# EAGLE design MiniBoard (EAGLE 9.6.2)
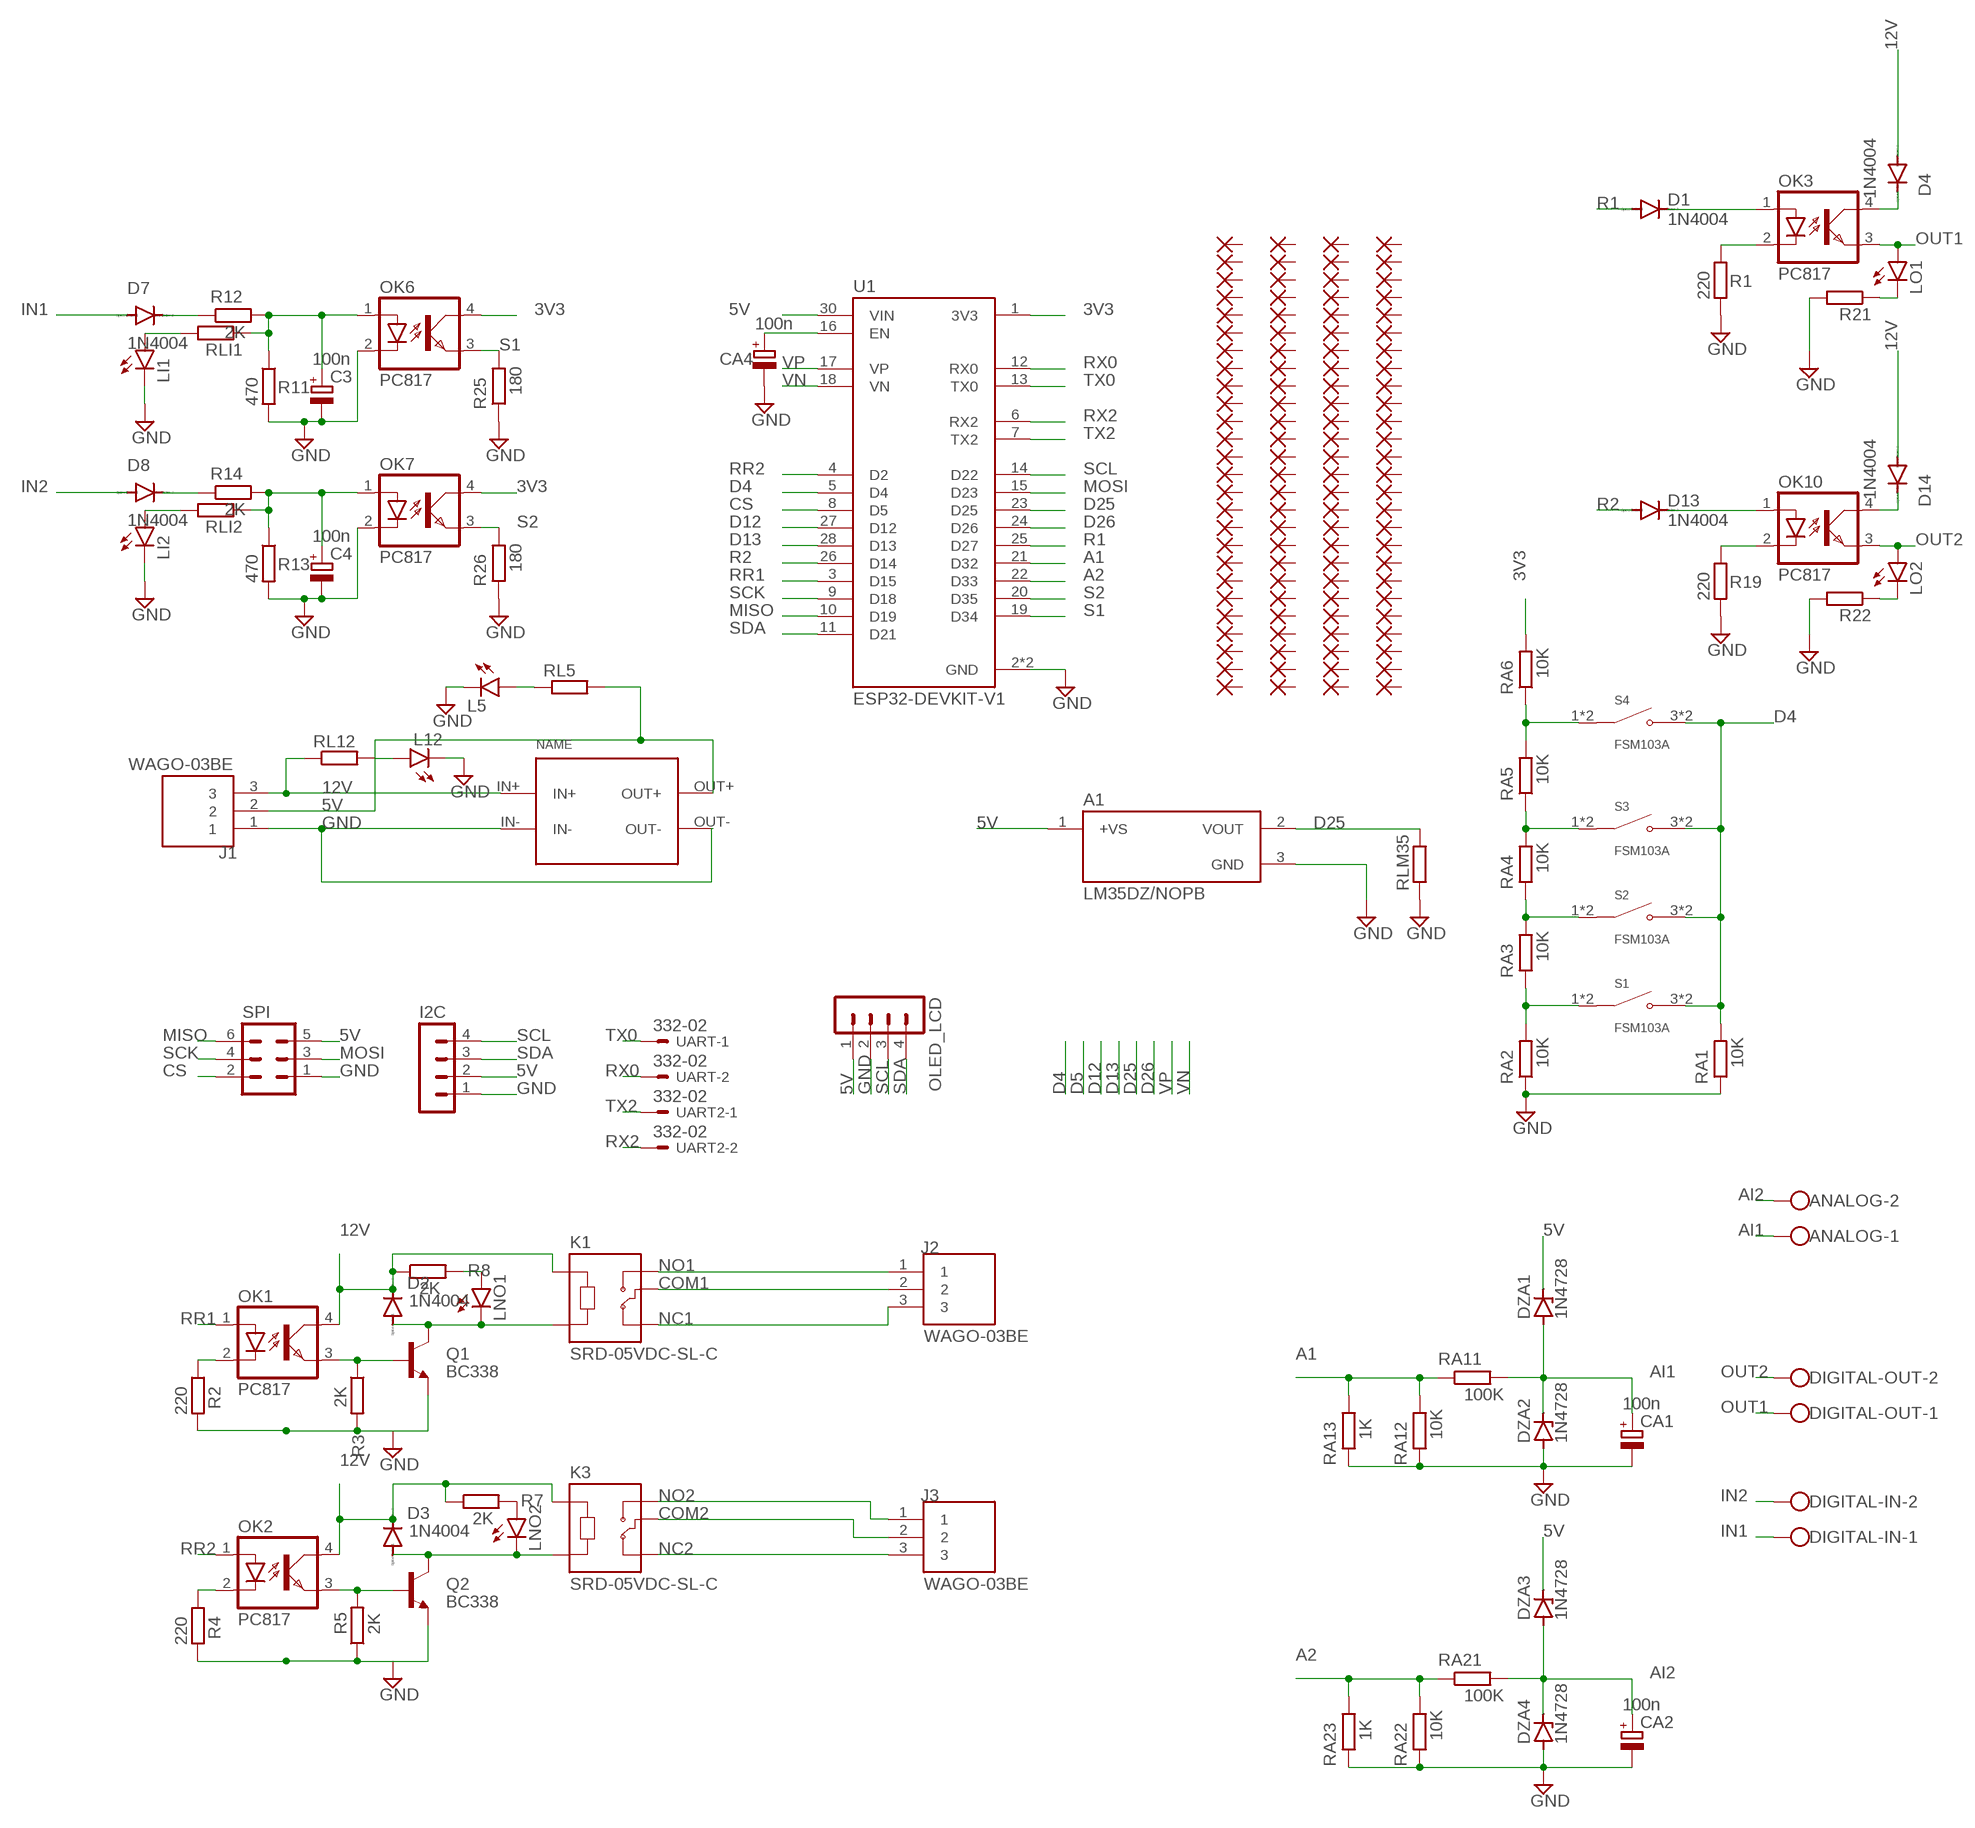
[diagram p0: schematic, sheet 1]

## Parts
A1  LM35DZ/NOPB  [TO92127P521H735-3]
ANALOG  W237-102  [W237-102]
C3  100n  CPOL-EUE5-6  [E5-6]
C4  100n  CPOL-EUE5-6  [E5-6]
CA1  100n  CPOL-EUE5-6  [E5-6]
CA2  100n  CPOL-EUE5-6  [E5-6]
CA4  100n  CPOL-EUE5-6  [E5-6]
D1  1N4004  [DO41-10]
D2  1N4004  [DO41-10]
D3  1N4004  [DO41-10]
D4  1N4004  [DO41-10]
D7  1N4004  [DO41-10]
D8  1N4004  [DO41-10]
D13  1N4004  [DO41-10]
D14  1N4004  [DO41-10]
DIGITAL-IN  W237-102  [W237-102]
DIGITAL-OUT  W237-102  [W237-102]
DZA1  1N4728  [DO41Z10]
DZA2  1N4728  [DO41Z10]
DZA3  1N4728  [DO41Z10]
DZA4  1N4728  [DO41Z10]
I2C  MA04-1  [MA04-1]
J1  WAGO-03BE  [CUI_TB006-508-03BE]
J2  WAGO-03BE  [CUI_TB006-508-03BE]
J3  WAGO-03BE  [CUI_TB006-508-03BE]
K1  SRD-05VDC-SL-C  [RELAY_SRD-05VDC-SL-C]
K3  SRD-05VDC-SL-C  [RELAY_SRD-05VDC-SL-C]
L5  LED3MM  [LED3MM]
L12  LED3MM  [LED3MM]
LI1  LED3MM  [LED3MM]
LI2  LED3MM  [LED3MM]
LNO1  LED3MM  [LED3MM]
LNO2  LED3MM  [LED3MM]
LO1  LED3MM  [LED3MM]
LO2  LED3MM  [LED3MM]
OK1  PC817  [DIL04]
OK2  PC817  [DIL04]
OK3  PC817  [DIL04]
OK6  PC817  [DIL04]
OK7  PC817  [DIL04]
OK10  PC817  [DIL04]
OLED_LCD  MA04-1  [MA04-1]
PAD1  WIREPAD1,6/0,9  [1,6/0,9]
PAD2  WIREPAD1,6/0,9  [1,6/0,9]
PAD3  WIREPAD1,6/0,9  [1,6/0,9]
PAD4  WIREPAD1,6/0,9  [1,6/0,9]
PAD5  WIREPAD1,6/0,9  [1,6/0,9]
PAD6  WIREPAD1,6/0,9  [1,6/0,9]
PAD7  WIREPAD1,6/0,9  [1,6/0,9]
PAD8  WIREPAD1,6/0,9  [1,6/0,9]
PAD9  WIREPAD1,6/0,9  [1,6/0,9]
PAD10  WIREPAD1,6/0,9  [1,6/0,9]
PAD11  WIREPAD1,6/0,9  [1,6/0,9]
PAD12  WIREPAD1,6/0,9  [1,6/0,9]
PAD13  WIREPAD1,6/0,9  [1,6/0,9]
PAD14  WIREPAD1,6/0,9  [1,6/0,9]
PAD15  WIREPAD1,6/0,9  [1,6/0,9]
PAD16  WIREPAD1,6/0,9  [1,6/0,9]
PAD17  WIREPAD1,6/0,9  [1,6/0,9]
PAD18  WIREPAD1,6/0,9  [1,6/0,9]
PAD19  WIREPAD1,6/0,9  [1,6/0,9]
PAD20  WIREPAD1,6/0,9  [1,6/0,9]
PAD21  WIREPAD1,6/0,9  [1,6/0,9]
PAD22  WIREPAD1,6/0,9  [1,6/0,9]
PAD23  WIREPAD1,6/0,9  [1,6/0,9]
PAD24  WIREPAD1,6/0,9  [1,6/0,9]
PAD25  WIREPAD1,6/0,9  [1,6/0,9]
PAD26  WIREPAD1,6/0,9  [1,6/0,9]
PAD27  WIREPAD1,6/0,9  [1,6/0,9]
PAD28  WIREPAD1,6/0,9  [1,6/0,9]
PAD29  WIREPAD1,6/0,9  [1,6/0,9]
PAD30  WIREPAD1,6/0,9  [1,6/0,9]
PAD31  WIREPAD1,6/0,9  [1,6/0,9]
PAD32  WIREPAD1,6/0,9  [1,6/0,9]
PAD33  WIREPAD1,6/0,9  [1,6/0,9]
PAD34  WIREPAD1,6/0,9  [1,6/0,9]
PAD35  WIREPAD1,6/0,9  [1,6/0,9]
PAD36  WIREPAD1,6/0,9  [1,6/0,9]
PAD37  WIREPAD1,6/0,9  [1,6/0,9]
PAD38  WIREPAD1,6/0,9  [1,6/0,9]
PAD39  WIREPAD1,6/0,9  [1,6/0,9]
PAD40  WIREPAD1,6/0,9  [1,6/0,9]
PAD41  WIREPAD1,6/0,9  [1,6/0,9]
PAD42  WIREPAD1,6/0,9  [1,6/0,9]
PAD43  WIREPAD1,6/0,9  [1,6/0,9]
PAD44  WIREPAD1,6/0,9  [1,6/0,9]
PAD45  WIREPAD1,6/0,9  [1,6/0,9]
PAD46  WIREPAD1,6/0,9  [1,6/0,9]
PAD47  WIREPAD1,6/0,9  [1,6/0,9]
PAD48  WIREPAD1,6/0,9  [1,6/0,9]
PAD49  WIREPAD1,6/0,9  [1,6/0,9]
PAD50  WIREPAD1,6/0,9  [1,6/0,9]
PAD51  WIREPAD1,6/0,9  [1,6/0,9]
PAD52  WIREPAD1,6/0,9  [1,6/0,9]
PAD53  WIREPAD1,6/0,9  [1,6/0,9]
PAD54  WIREPAD1,6/0,9  [1,6/0,9]
PAD55  WIREPAD1,6/0,9  [1,6/0,9]
PAD56  WIREPAD1,6/0,9  [1,6/0,9]
PAD57  WIREPAD1,6/0,9  [1,6/0,9]
PAD58  WIREPAD1,6/0,9  [1,6/0,9]
PAD59  WIREPAD1,6/0,9  [1,6/0,9]
PAD60  WIREPAD1,6/0,9  [1,6/0,9]
PAD61  WIREPAD1,6/0,9  [1,6/0,9]
PAD62  WIREPAD1,6/0,9  [1,6/0,9]
PAD63  WIREPAD1,6/0,9  [1,6/0,9]
PAD64  WIREPAD1,6/0,9  [1,6/0,9]
PAD65  WIREPAD1,6/0,9  [1,6/0,9]
PAD66  WIREPAD1,6/0,9  [1,6/0,9]
PAD67  WIREPAD1,6/0,9  [1,6/0,9]
PAD68  WIREPAD1,6/0,9  [1,6/0,9]
PAD69  WIREPAD1,6/0,9  [1,6/0,9]
PAD70  WIREPAD1,6/0,9  [1,6/0,9]
PAD71  WIREPAD1,6/0,9  [1,6/0,9]
PAD72  WIREPAD1,6/0,9  [1,6/0,9]
PAD73  WIREPAD1,6/0,9  [1,6/0,9]
PAD74  WIREPAD1,6/0,9  [1,6/0,9]
PAD75  WIREPAD1,6/0,9  [1,6/0,9]
PAD76  WIREPAD1,6/0,9  [1,6/0,9]
PAD77  WIREPAD1,6/0,9  [1,6/0,9]
PAD78  WIREPAD1,6/0,9  [1,6/0,9]
PAD79  WIREPAD1,6/0,9  [1,6/0,9]
PAD80  WIREPAD1,6/0,9  [1,6/0,9]
PAD81  WIREPAD1,6/0,9  [1,6/0,9]
PAD82  WIREPAD1,6/0,9  [1,6/0,9]
PAD83  WIREPAD1,6/0,9  [1,6/0,9]
PAD84  WIREPAD1,6/0,9  [1,6/0,9]
PAD85  WIREPAD1,6/0,9  [1,6/0,9]
PAD86  WIREPAD1,6/0,9  [1,6/0,9]
PAD87  WIREPAD1,6/0,9  [1,6/0,9]
PAD88  WIREPAD1,6/0,9  [1,6/0,9]
PAD89  WIREPAD1,6/0,9  [1,6/0,9]
PAD90  WIREPAD1,6/0,9  [1,6/0,9]
PAD91  WIREPAD1,6/0,9  [1,6/0,9]
PAD92  WIREPAD1,6/0,9  [1,6/0,9]
PAD93  WIREPAD1,6/0,9  [1,6/0,9]
PAD94  WIREPAD1,6/0,9  [1,6/0,9]
PAD95  WIREPAD1,6/0,9  [1,6/0,9]
PAD96  WIREPAD1,6/0,9  [1,6/0,9]
PAD97  WIREPAD1,6/0,9  [1,6/0,9]
PAD98  WIREPAD1,6/0,9  [1,6/0,9]
PAD99  WIREPAD1,6/0,9  [1,6/0,9]
PAD100  WIREPAD1,6/0,9  [1,6/0,9]
PAD101  WIREPAD1,6/0,9  [1,6/0,9]
PAD102  WIREPAD1,6/0,9  [1,6/0,9]
PAD103  WIREPAD1,6/0,9  [1,6/0,9]
PAD104  WIREPAD1,6/0,9  [1,6/0,9]
Q1  BC338  [TO92-EBC]
Q2  BC338  [TO92-EBC]
R1  220  R-EU_0309/12  [0309/12]
R2  220  R-EU_0309/12  [0309/12]
R3  2K  R-EU_0309/12  [0309/12]
R4  220  R-EU_0309/12  [0309/12]
R5  2K  R-EU_0309/12  [0309/12]
R7  2K  R-EU_0309/12  [0309/12]
R8  2K  R-EU_0309/12  [0309/12]
R11  470  R-EU_0309/12  [0309/12]
R12  2K  R-EU_0309/12  [0309/12]
R13  470  R-EU_0309/12  [0309/12]
R14  2K  R-EU_0309/12  [0309/12]
R19  220  R-EU_0309/12  [0309/12]
R21  R-EU_0309/12  [0309/12]
R22  R-EU_0309/12  [0309/12]
R25  180  R-EU_0309/12  [0309/12]
R26  180  R-EU_0309/12  [0309/12]
RA1  10K  R-EU_0309/12  [0309/12]
RA2  10K  R-EU_0309/12  [0309/12]
RA3  10K  R-EU_0309/12  [0309/12]
RA4  10K  R-EU_0309/12  [0309/12]
RA5  10K  R-EU_0309/12  [0309/12]
RA6  10K  R-EU_0309/12  [0309/12]
RA11  100K  R-EU_0309/12  [0309/12]
RA12  10K  R-EU_0309/12  [0309/12]
RA13  1K  R-EU_0309/12  [0309/12]
RA21  100K  R-EU_0309/12  [0309/12]
RA22  10K  R-EU_0309/12  [0309/12]
RA23  1K  R-EU_0309/12  [0309/12]
RL5  R-EU_0309/12  [0309/12]
RL12  R-EU_0309/12  [0309/12]
RLI1  R-EU_0309/12  [0309/12]
RLI2  R-EU_0309/12  [0309/12]
RLM35  R-EU_0309/12  [0309/12]
S1  FSM103A  [SW_1571627-1]
S2  FSM103A  [SW_1571627-1]
S3  FSM103A  [SW_1571627-1]
S4  FSM103A  [SW_1571627-1]
SPI  MA03-2  [MA03-2]
U1  ESP32-DEVKIT-V1  [MODULE_ESP32_DEVKIT_V1]
U$1  CP8-ADJ  [CP8-ADJ]
UART  332-02  [332-02]
UART2  332-02  [332-02]

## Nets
3V3: OK6.4(COL) OK7.4(COL) RA6.2 U1.1(3V3)
5V: A1.1(+VS) DZA1.C DZA3.C I2C.2 J1.2 OLED_LCD.1 RL5.2 SPI.5 U1.30(VIN) U$1.OUT+
12V: D2.C D3.C D4.A D14.A J1.3 K1.A1 K3.A1 OK1.4(COL) OK2.4(COL) R7.1 R8.1 RL12.1 U$1.IN+
A1: RA11.1 RA12.2 RA13.2 U1.21(D32)
A2: RA21.1 RA22.2 RA23.2 U1.22(D33)
AI1: ANALOG.1 CA1.+ DZA1.A DZA2.C RA11.2
AI2: ANALOG.2 CA2.+ DZA3.A DZA4.C RA21.2
COM1: J2.2 K1.COM
COM2: J3.2 K3.COM
CS: SPI.2 U1.8(D5)
D4: RA1.2 S1.3(NO) S1.4(NO) S2.3(NO) S2.4(NO) S3.3(NO) S3.4(NO) S4.3(NO) S4.4(NO) U1.5(D4)
D12: U1.27(D12)
D13: U1.28(D13)
D25: A1.2(VOUT) RLM35.2 U1.23(D25)
D26: U1.24(D26)
GND: A1.3(GND) C3.- C4.- CA1.- CA2.- CA4.- DZA2.A DZA4.A I2C.1 J1.1 L5.K(C) L12.K(C) LI1.K(C) LI2.K(C) OK6.2(C) OK7.2(C) OLED_LCD.2 Q1.E Q2.E R1.2 R2.2 R3.2 R4.2 R5.1 R11.2 R13.2 R19.2 R21.2 R22.2 R25.1 R26.1 RA1.1 RA2.1 RA12.1 RA13.1 RA22.1 RA23.1 RLM35.1 SPI.1 U1.2(GND) U1.29(GND) U$1.IN- U$1.OUT-
IN1: D7.A DIGITAL-IN.1
IN2: D8.A DIGITAL-IN.2
MISO: SPI.6 U1.10(D19)
MOSI: SPI.3 U1.15(D23)
N$1: OK2.2(C) R4.1
N$2: OK1.2(C) R2.1
N$3: OK1.3(EMIT) Q1.B R3.1
N$4: D3.A K3.A2 LNO2.K(C) Q2.C
N$5: RA4.2 RA5.1 S3.1(COM) S3.2(COM)
N$6: OK2.3(EMIT) Q2.B R5.2
N$7: LNO2.A R7.2
N$8: RA3.2 RA4.1 S2.1(COM) S2.2(COM)
N$9: RA2.2 RA3.1 S1.1(COM) S1.2(COM)
N$10: LNO1.A R8.2
N$11: D2.A K1.A2 LNO1.K(C) Q1.C
N$14: L12.A RL12.2
N$15: D1.C OK3.1(A)
N$16: OK3.2(C) R1.1
N$18: D4.C OK3.4(COL)
N$19: C3.+ OK6.1(A) R11.1 R12.2 RLI1.1
N$20: D7.C R12.1
N$21: C4.+ OK7.1(A) R13.1 R14.2 RLI2.1
N$22: D8.C R14.1
N$23: L5.A RL5.1
N$24: LI2.A RLI2.2
N$25: CA4.+ U1.16(EN)
N$26: D13.C OK10.1(A)
N$27: OK10.2(C) R19.1
N$29: LI1.A RLI1.2
N$30: LO1.K(C) R21.1
N$31: LO2.K(C) R22.1
N$32: RA5.2 RA6.1 S4.1(COM) S4.2(COM)
N$52: D14.C OK10.4(COL)
NC1: J2.3 K1.NC
NC2: J3.3 K3.NC
NO1: J2.1 K1.NO
NO2: J3.1 K3.NO
OUT1: DIGITAL-OUT.1 LO1.A OK3.3(EMIT)
OUT2: DIGITAL-OUT.2 LO2.A OK10.3(EMIT)
R1: D1.A U1.25(D27)
R2: D13.A U1.26(D14)
RR1: OK1.1(A) U1.3(D15)
RR2: OK2.1(A) U1.4(D2)
RX0: U1.12(RX0) UART.2
RX2: U1.6(RX2) UART2.2
S1: OK6.3(EMIT) R25.2 U1.19(D34)
S2: OK7.3(EMIT) R26.2 U1.20(D35)
SCK: SPI.4 U1.9(D18)
SCL: I2C.4 OLED_LCD.3 U1.14(D22)
SDA: I2C.3 OLED_LCD.4 U1.11(D21)
TX0: U1.13(TX0) UART.1
TX2: U1.7(TX2) UART2.1
VN: U1.18(VN)
VP: U1.17(VP)
Unconnected: PAD1.1(P) PAD2.1(P) PAD3.1(P) PAD4.1(P) PAD5.1(P) PAD6.1(P) PAD7.1(P) PAD8.1(P) PAD9.1(P) PAD10.1(P) PAD11.1(P) PAD12.1(P) PAD13.1(P) PAD14.1(P) PAD15.1(P) PAD16.1(P) PAD17.1(P) PAD18.1(P) PAD19.1(P) PAD20.1(P) PAD21.1(P) PAD22.1(P) PAD23.1(P) PAD24.1(P) PAD25.1(P) PAD26.1(P) PAD27.1(P) PAD28.1(P) PAD29.1(P) PAD30.1(P) PAD31.1(P) PAD32.1(P) PAD33.1(P) PAD34.1(P) PAD35.1(P) PAD36.1(P) PAD37.1(P) PAD38.1(P) PAD39.1(P) PAD40.1(P) PAD41.1(P) PAD42.1(P) PAD43.1(P) PAD44.1(P) PAD45.1(P) PAD46.1(P) PAD47.1(P) PAD48.1(P) PAD49.1(P) PAD50.1(P) PAD51.1(P) PAD52.1(P) PAD53.1(P) PAD54.1(P) PAD55.1(P) PAD56.1(P) PAD57.1(P) PAD58.1(P) PAD59.1(P) PAD60.1(P) PAD61.1(P) PAD62.1(P) PAD63.1(P) PAD64.1(P) PAD65.1(P) PAD66.1(P) PAD67.1(P) PAD68.1(P) PAD69.1(P) PAD70.1(P) PAD71.1(P) PAD72.1(P) PAD73.1(P) PAD74.1(P) PAD75.1(P) PAD76.1(P) PAD77.1(P) PAD78.1(P) PAD79.1(P) PAD80.1(P) PAD81.1(P) PAD82.1(P) PAD83.1(P) PAD84.1(P) PAD85.1(P) PAD86.1(P) PAD87.1(P) PAD88.1(P) PAD89.1(P) PAD90.1(P) PAD91.1(P) PAD92.1(P) PAD93.1(P) PAD94.1(P) PAD95.1(P) PAD96.1(P) PAD97.1(P) PAD98.1(P) PAD99.1(P) PAD100.1(P) PAD101.1(P) PAD102.1(P) PAD103.1(P) PAD104.1(P)

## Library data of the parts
A1 = LM35DZ_NOPB:LM35DZ/NOPB; CHECK_PRICES: https://www.snapeda.com/parts/LM35DZ/NOPB/Texas+Instruments/view-part/?ref=eda; DESCRIPTION: 1C high voltage analog temperature sensor, 10 mV/C; DIGIKEY_PART_NUMBER: LM35DZ/NOPB-ND; MF: Texas; MP: LM35DZ/NOPB; PACKAGE: None; SNAPEDA_LINK: https://www.snapeda.com/parts/LM35DZ/NOPB/Texas+Instruments/view-part/?ref=snap
ANALOG DIGITAL-IN DIGITAL-OUT = con-wago-500:W237-102: WAGO SCREW CLAMP; MPN: 237-102; OC_FARNELL: unknown; OC_NEWARK: 70K9898
C3 C4 CA1 CA2 CA4 = rcl-ws:CPOL-EU: POLARIZED CAPACITOR, European symbol; SPICEPREFIX: C
D1-D4 D7 D8 D13 D14 = diode:1N4004: DIODE
DZA1-DZA4 = diode-ws:1N4728: Z DIODE
I2C OLED_LCD = con-lstb:MA04-1: PIN HEADER; OC_FARNELL: unknown; OC_NEWARK: unknown
J1-J3 = TB006-508-03BE:WAGO-03BE: Check availability; AVAILABILITY: In Stock; CHECK_PRICES: https://www.snapeda.com/parts/TB006-508-03BE/Same+Sky/view-part/?ref=eda; DESCRIPTION: 2~24 Poles, Screw Type, Horizontal, 5.08 Pitch, 26~14 (AWG), Terminal Block Connector; MF: Same Sky; MP: TB006-508-03BE; PACKAGE: None; PRICE: None; SNAPEDA_LINK: https://www.snapeda.com/parts/TB006-508-03BE/Same+Sky/view-part/?ref=snap
K1 K3 = SRD-05VDC-SL-C:SRD-05VDC-SL-C: 5V Trigger Relay Module For Arduino And Raspberry Pi 5V Trigger Relay Module For Arduino And Raspberry Pi Check availability; AVAILABILITY: In Stock; CHECK_PRICES: https://www.snapeda.com/parts/SRD-05VDC-SL-C/Songle+Relay/view-part/?ref=eda; DESCRIPTION: 5V Trigger Relay Module For Arduino And Raspberry Pi 5V Trigger Relay Module For Arduino And Raspberry Pi; MF: Songle Relay; MP: SRD-05VDC-SL-C; PACKAGE: NON STANDARD-5 Songle Relay; PRICE: None; SNAPEDA_LINK: https://www.snapeda.com/parts/SRD-05VDC-SL-C/Songle+Relay/view-part/?ref=snap
L5 L12 LI1 LI2 LNO1 LNO2 LO1 LO2 = led_WS:LED: LED
OK1-OK3 OK6 OK7 OK10 = optocoupler:PC817: SHARP OPTO COUPLER; MPN: PC817X4J000F; OC_FARNELL: 9707727; OC_NEWARK: 97K7059
PAD1-PAD104 = wirepad-ws:WIREPAD: Wire PAD connect wire on PCB
Q1 Q2 = transistor-npn:BC338*: NPN Transistor
R1-R5 R7 R8 R11-R14 R19 R21 R22 R25 R26 RA1-RA6 RA11-RA13 RA21-RA23 RL5 RL12 RLI1 RLI2 RLM35 = rcl-ws:R-EU_: RESISTOR, European symbol; SPICEPREFIX: R
S1-S4 = FSM103A:FSM103A: Alcoswitch FSM100-104, Tactile Switches, Round Actuator Style, Operating Function NO, Brass Contact Base Material Check availability; AVAILABILITY: In Stock; CHECK_PRICES: https://www.snapeda.com/parts/FSM103A/TE+Connectivity+ALCOSWITCH+Switches/view-part/?ref=eda; COMMENT: 1571627-1; DESCRIPTION: Alcoswitch, Tactile switch,PCB,SPST,red actuator | TE Connectivity FSM103A; MF: TE Connectivity; MP: FSM103A; PACKAGE: None; PRICE: None; SNAPEDA_LINK: https://www.snapeda.com/parts/FSM103A/TE+Connectivity+ALCOSWITCH+Switches/view-part/?ref=snap
SPI = con-lstb-ws:MA03-2: PIN HEADER; OC_FARNELL: unknown; OC_NEWARK: unknown
U1 = ESP32-DEVKIT-V1:ESP32-DEVKIT-V1: Dual core, Wi-Fi: 2.4 GHz up to 150 Mbits/s,BLE (Bluetooth Low Energy) and legacy Bluetooth, 32 bits, Up to 240 MHz Check availability; AVAILABILITY: Not in stock; CHECK_PRICES: https://www.snapeda.com/parts/ESP32-DEVKIT-V1/Do+it/view-part/?ref=eda; DESCRIPTION: Dual core, Wi-Fi: 2.4 GHz up to 150 Mbits/s,BLE (Bluetooth Low Energy) and legacy Bluetooth, 32 bits, Up to 240 MHz; MF: Do it; MP: ESP32-DEVKIT-V1; PACKAGE: None; PRICE: None; SNAPEDA_LINK: https://www.snapeda.com/parts/ESP32-DEVKIT-V1/Do+it/view-part/?ref=snap
U$1 = userlib:CP8-ADJ: Voltage regulator IN: 7-35V OUT: ADJ
UART UART2 = con-garry-ws:332-02: 2 Pin - 2mm Dual Row

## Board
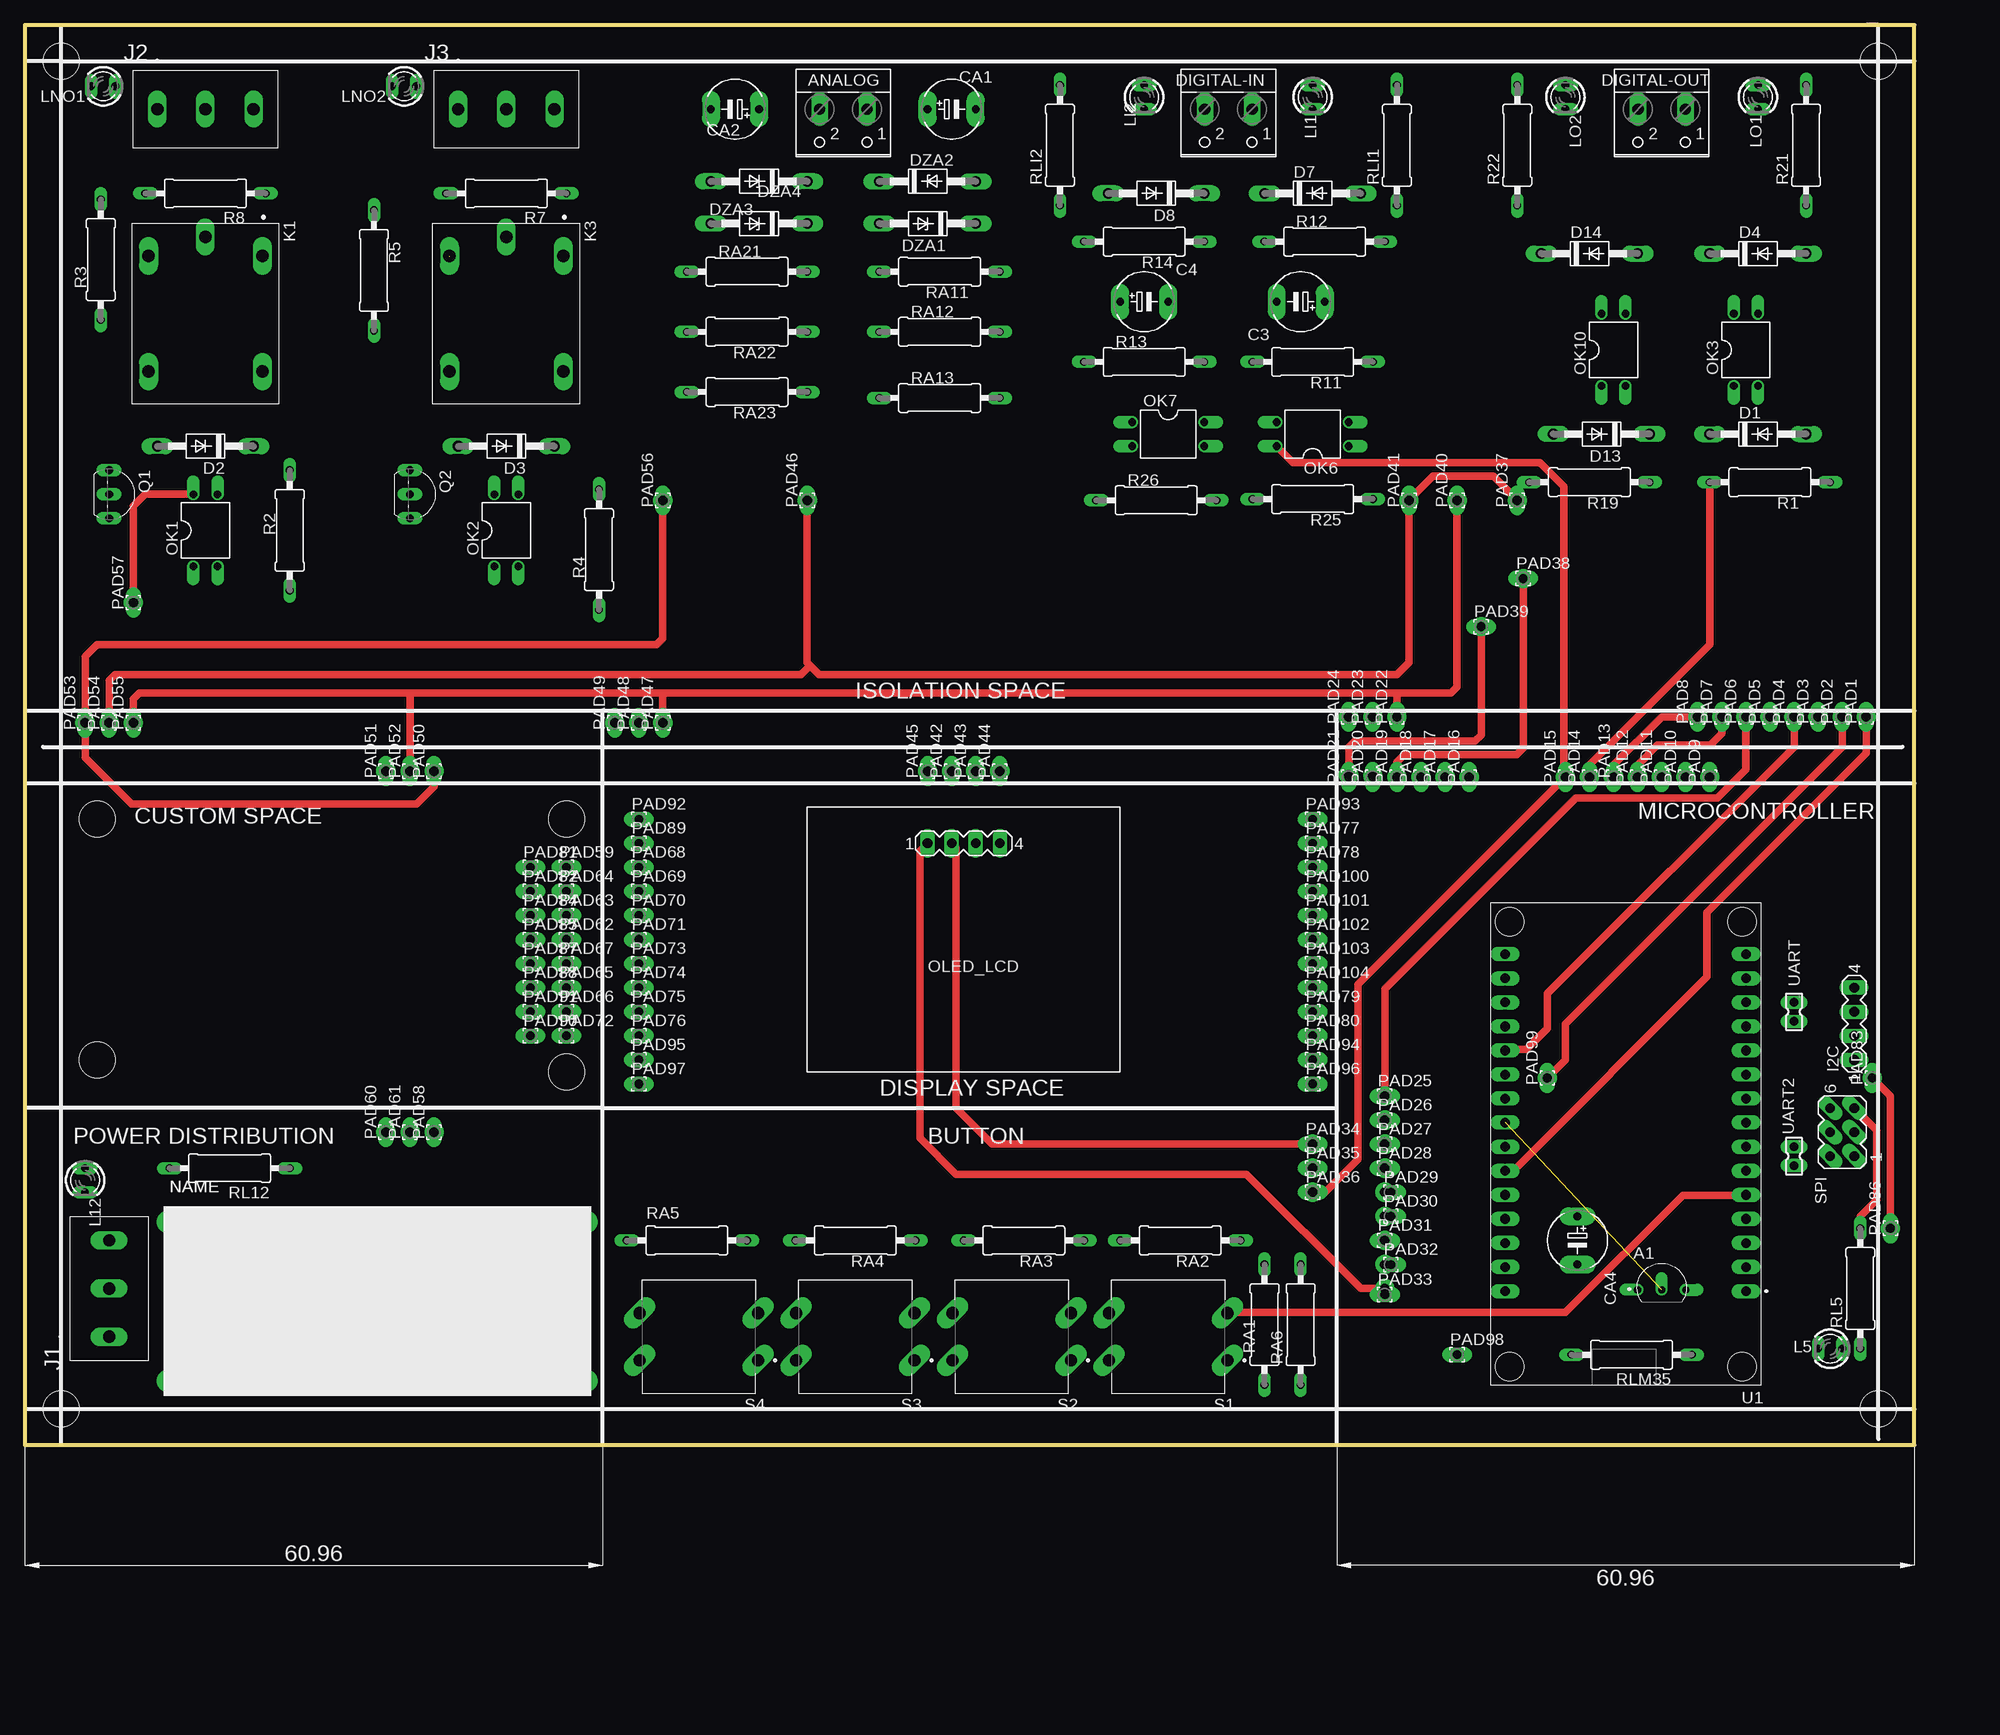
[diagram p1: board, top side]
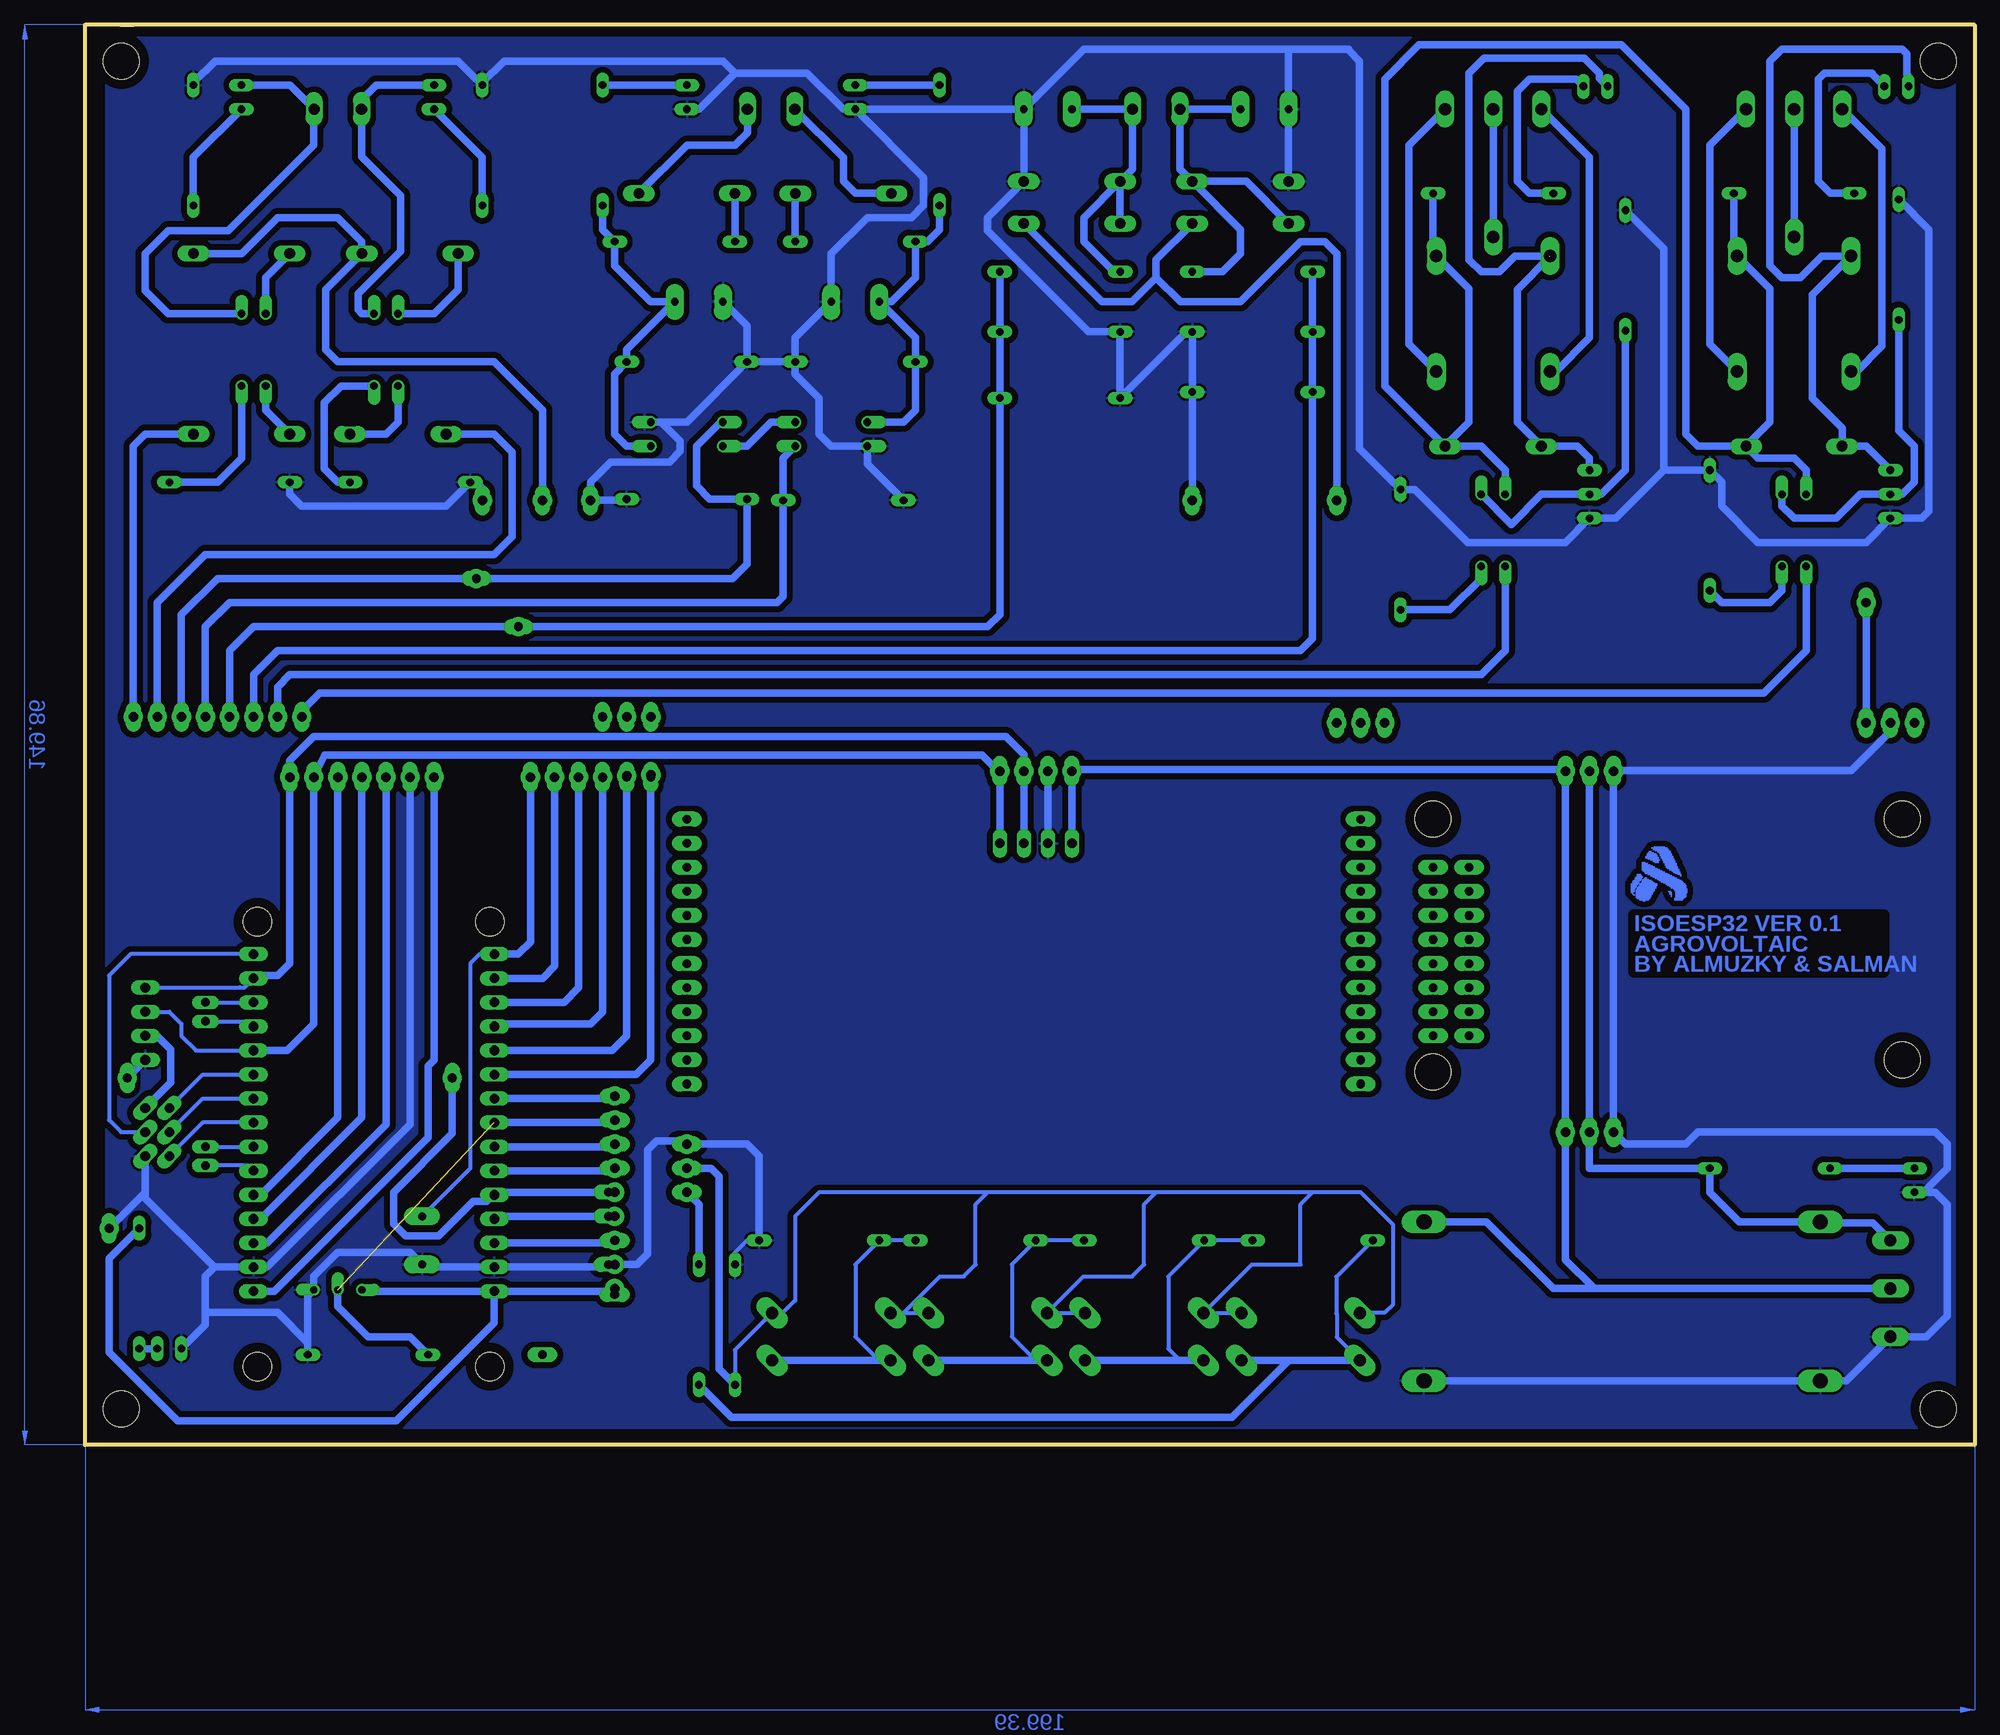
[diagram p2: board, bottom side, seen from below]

Size 199.39 x 149.86 mm. Coordinates in mm from the lower left corner, seen from the top.
Outline: 195.58,149.86 194.31,149.86
Outline: 0,0 199.39,0 199.39,149.86 0,149.86 0,0
Copper layers (1*16): Top 0.035mm / dielectric 1.5mm / Bottom 0.035mm
Design rules "default *": minimum track width 16mil, minimum drill 0.35mm, track to track 24mil, track to pad 24mil, pad to pad 24mil, via to via 6mil, smd to smd 6mil, copper to edge 40mil, drill to drill 6mil, minimum pad ring 10mil, minimum via ring 8mil, stop-mask expansion 4mil, vias tented up to drill 0mil, thermal gap 10mil
Holes 3.81 mm at 195.58,146.05 195.58,3.81 3.81,3.81 3.81,146.05 57.15,66.04 7.62,66.04 7.62,40.64 57.15,39.37

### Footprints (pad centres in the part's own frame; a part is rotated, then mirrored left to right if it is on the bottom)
TO92127P521H735-3 = drill 0.75 pad 0.813 offset: 1 -2.54,-0.775; 2 0,-0.775; 3 2.54,-0.775
W237-102 = drill 1.194 long: 1 -2.5,-1.27; 2 2.5,-1.27
E5-6 = drill 0.813 pad 1.905 long: + -2.54,0; - 2.54,0
DO41-10 = drill 1.118 long: A 5.08,0; C -5.08,0
DO41Z10 = drill 1.118 long: A 5.08,0; C -5.08,0
MA04-1 = drill 1.016 long: 1 -3.81,0; 2 -1.27,0; 3 1.27,0; 4 3.81,0
CUI_TB006-508-03BE = drill 1.3 long: 1 0,0; 2 5.08,0; 3 10.16,0
RELAY_SRD-05VDC-SL-C = drill 1.32 long: A1 -6.1,6; A2 -6.1,-6; NC 6.1,6; NO 6.1,-6 | drill 1.29 long: COM -8.1,0
LED3MM = drill 0.813 long: A -1.27,0; K 1.27,0
DIL04 = drill 0.813 offset: 1 -1.27,-3.81; 2 1.27,-3.81; 3 1.27,3.81; 4 -1.27,3.81
1,6/0,9 = drill 0.914 pad 1.6 long: 1 0,0
TO92-EBC = drill 0.813 long: B 0,-1.27; C -2.54,-1.27; E 2.54,-1.27
0309/12 = drill 0.813 long: 1 -6.35,0; 2 6.35,0
SW_1571627-1 = drill 1.3 long: 1 -6.25,2.5; 2 6.25,2.5; 3 -6.25,-2.5; 4 6.25,-2.5
MA03-2 = drill 1.016 pad 1.016 long: 1 -2.54,-1.27; 2 -2.54,1.27; 3 0,-1.27; 4 0,1.27; 5 2.54,-1.27; 6 2.54,1.27
MODULE_ESP32_DEVKIT_V1 = drill 1.02 pad 1.27 long: 1 -12.7,15.515; 2 -12.7,12.975; 3 -12.7,10.435; 4 -12.7,7.895; 5 -12.7,5.355; 6 -12.7,2.815; 7 -12.7,0.275; 8 -12.7,-2.265; 9 -12.7,-4.805; 10 -12.7,-7.345; 11 -12.7,-9.885; 12 -12.7,-12.425; 13 -12.7,-14.965; 14 -12.7,-17.505; 15 -12.7,-20.045; 16 12.7,-20.045; 17 12.7,-17.505; 18 12.7,-14.965; 19 12.7,-12.425; 20 12.7,-9.885; 21 12.7,-7.345; 22 12.7,-4.805; 23 12.7,-2.265; 24 12.7,0.275; 25 12.7,2.815; 26 12.7,5.355; 27 12.7,7.895; 28 12.7,10.435; 29 12.7,12.975; 30 12.7,15.515 | hole 3: -12.28,-23.475; 12.23,-23.475; 12.23,23.475; -12.28,23.475
CP8-ADJ = drill 1.6 long: IN+ -21.81,7.05; IN- -21.81,-9.75; OUT+ 19.99,7.05; OUT- 19.99,-9.75
332-02 = drill 0.9 pad 1.016 long: 1 0,-1; 2 0,1

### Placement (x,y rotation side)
A1  172.72,17.14 0 top
ANALOG  86.36,139.7 180 top
C3  134.62,120.65 180 top
C4  118.11,120.65 0 top
CA1  97.79,140.97 0 top
CA2  74.93,140.97 180 top
CA4  163.83,21.59 270 top
D1  182.88,106.68 0 top
D2  19.05,105.41 180 top
D3  50.8,105.41 180 top
D4  182.88,125.73 0 top
D7  135.89,132.08 0 top
D8  119.38,132.08 180 top
D13  166.37,106.68 180 top
D14  165.1,125.73 0 top
DIGITAL-IN  127,139.7 180 top
DIGITAL-OUT  172.72,139.7 180 top
DZA1  95.25,128.91 180 top
DZA2  95.25,133.35 0 top
DZA3  77.47,128.91 180 top
DZA4  77.47,133.35 180 top
I2C  193.04,44.45 90 top
J1  8.89,11.43 90 top
J2  13.97,140.97 0 top
J3  45.72,140.97 0 top
K1  19.05,119.38 270 top
K3  50.8,119.38 270 top
L5  190.5,10.16 180 top
L12  6.35,27.94 270 top
LI1  135.89,142.24 270 top
LI2  118.11,142.24 270 top
LNO1  8.26,143.38 180 top
LNO2  40.01,143.38 180 top
LO1  182.88,142.24 270 top
LO2  162.56,142.24 270 top
OK1  19.05,96.52 0 top
OK2  50.8,96.52 0 top
OK3  181.61,115.57 0 top
OK6  135.89,106.68 90 top
OK7  120.65,106.68 270 top
OK10  167.64,115.57 0 top
OLED_LCD  99.06,63.5 0 top
PAD1  194.31,76.83 90 top
PAD2  191.77,76.83 90 top
PAD3  189.23,76.83 90 top
PAD4  186.69,76.83 90 top
PAD5  184.15,76.83 90 top
PAD6  181.61,76.83 90 top
PAD7  179.07,76.83 90 top
PAD8  176.53,76.83 90 top
PAD9  177.8,70.48 90 top
PAD10  175.26,70.48 90 top
PAD11  172.72,70.48 90 top
PAD12  170.18,70.48 90 top
PAD13  167.64,70.48 90 top
PAD14  165.1,70.48 90 top
PAD15  162.56,70.48 90 top
PAD16  152.4,70.48 90 top
PAD17  149.86,70.48 90 top
PAD18  147.32,70.48 90 top
PAD19  144.78,70.48 90 top
PAD20  142.24,70.48 90 top
PAD21  139.7,70.48 90 top
PAD22  144.78,76.83 90 top
PAD23  142.24,76.83 90 top
PAD24  139.7,76.83 90 top
PAD25  143.51,36.83 0 top
PAD26  143.51,34.29 0 top
PAD27  143.51,31.75 0 top
PAD28  143.51,29.21 0 top
PAD29  144.15,26.67 0 top
PAD30  144.15,24.13 0 top
PAD31  143.51,21.59 0 top
PAD32  144.15,19.05 0 top
PAD33  143.51,15.88 0 top
PAD34  135.89,31.75 0 top
PAD35  135.89,29.21 0 top
PAD36  135.89,26.67 0 top
PAD37  157.48,99.69 90 top
PAD38  158.12,91.44 0 top
PAD39  153.67,86.36 0 top
PAD40  151.13,99.69 90 top
PAD41  146.05,99.69 90 top
PAD42  97.79,71.12 90 top
PAD43  100.33,71.12 90 top
PAD44  102.87,71.12 90 top
PAD45  95.25,71.12 90 top
PAD46  82.55,99.69 90 top
PAD47  67.31,76.2 90 top
PAD48  64.77,76.2 90 top
PAD49  62.23,76.2 90 top
PAD50  43.18,71.12 90 top
PAD51  38.1,71.12 90 top
PAD52  40.64,71.12 90 top
PAD53  6.35,76.2 90 top
PAD54  8.89,76.2 90 top
PAD55  11.43,76.2 90 top
PAD56  67.31,99.69 90 top
PAD57  11.43,88.9 90 top
PAD58  43.18,33.02 90 top
PAD59  57.15,60.96 0 top
PAD60  38.1,33.02 90 top
PAD61  40.64,33.02 90 top
PAD62  57.15,53.34 0 top
PAD63  57.15,55.88 0 top
PAD64  57.15,58.42 0 top
PAD65  57.15,48.26 0 top
PAD66  57.15,45.72 0 top
PAD67  57.15,50.8 0 top
PAD68  64.77,60.96 0 top
PAD69  64.77,58.42 0 top
PAD70  64.77,55.88 0 top
PAD71  64.77,53.34 0 top
PAD72  57.15,43.18 0 top
PAD73  64.77,50.8 0 top
PAD74  64.77,48.26 0 top
PAD75  64.77,45.72 0 top
PAD76  64.77,43.18 0 top
PAD77  135.89,63.5 0 top
PAD78  135.89,60.96 0 top
PAD79  135.89,45.72 0 top
PAD80  135.89,43.18 0 top
PAD81  53.34,60.96 0 top
PAD82  53.34,58.42 0 top
PAD83  194.94,38.73 90 top
PAD84  53.34,55.88 0 top
PAD85  53.34,53.34 0 top
PAD86  196.85,22.86 90 top
PAD87  53.34,50.8 0 top
PAD88  53.34,48.26 0 top
PAD89  64.77,63.5 0 top
PAD90  53.34,43.18 0 top
PAD91  53.34,45.72 0 top
PAD92  64.77,66.04 0 top
PAD93  135.89,66.04 0 top
PAD94  135.89,40.64 0 top
PAD95  64.77,40.64 0 top
PAD96  135.89,38.1 0 top
PAD97  64.77,38.1 0 top
PAD98  151.13,9.53 0 top
PAD99  160.66,38.73 90 top
PAD100  135.89,58.42 0 top
PAD101  135.89,55.88 0 top
PAD102  135.89,53.34 0 top
PAD103  135.89,50.8 0 top
PAD104  135.89,48.26 0 top
Q1  10.16,100.33 270 top
Q2  41.91,100.33 270 top
R1  184.15,101.6 180 top
R2  27.94,96.52 90 top
R3  8,125.09 90 top
R4  60.58,94.49 90 top
R5  36.83,123.95 270 top
R7  50.8,132.08 180 top
R8  19.05,132.08 180 top
R11  135.89,114.3 180 top
R12  137.16,127 0 top
R13  118.11,114.3 0 top
R14  118.11,127 180 top
R19  165.1,101.6 180 top
R21  187.96,137.16 90 top
R22  157.48,137.16 90 top
R25  135.89,99.82 180 top
R26  119.38,99.69 0 top
RA1  130.81,12.7 270 top
RA2  121.92,21.59 180 top
RA3  105.41,21.59 180 top
RA4  87.63,21.59 180 top
RA5  69.85,21.59 180 top
RA6  134.62,12.7 90 top
RA11  96.52,123.83 180 top
RA12  96.52,117.47 0 top
RA13  96.52,110.49 0 top
RA21  76.2,123.83 0 top
RA22  76.2,117.47 180 top
RA23  76.2,111.12 180 top
RL5  193.68,16.51 90 top
RL12  21.59,29.21 180 top
RLI1  144.78,137.16 90 top
RLI2  109.22,137.16 90 top
RLM35  169.54,9.53 180 top
S1  120.65,11.43 180 top
S2  104.14,11.43 180 top
S3  87.63,11.43 180 top
S4  71.12,11.43 180 top
SPI  191.77,33.02 90 top
U1  168.91,31.75 180 top
U$1  38.1,16.51 0 top
UART  186.69,45.72 180 top
UART2  186.69,30.48 180 top

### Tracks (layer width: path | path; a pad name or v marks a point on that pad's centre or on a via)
3V3  (via drill 1 pad 2.03)
  Top 0.813: v135.89,26.67 137.16,26.67 140.65,30.16 140.65,48.58 v162.56,70.48 162.4,70.8 162.4,101.12 159.86,103.66 133.83,103.66 OK6.4
  Bottom 0.813: RA6.2 134.62,25.4 v135.89,26.67 | OK7.4 127,107.95 129.54,105.41 OK6.4 | U1.1 179.42,16.23 163.19,32.46 163.19,40.01 162.56,40.64 v162.56,70.48
5V  (via drill 1 pad 2.03)
  Top 0.813: v67.31,99.69 67.31,85.09 66.67,84.45 7.62,84.45 6.35,83.19 v6.35,76.2 6.35,72.55 11.27,67.63 41.34,67.63 43.18,69.47 v43.18,71.12 | SPI.5 195.42,33.18 195.42,25.88 193.68,24.13 RL5.2 | v143.51,16.51 140.97,16.51 128.91,28.57 98.27,28.57 94.46,32.38 94.46,62.71 OLED_LCD.1
  Bottom 0.406: 152.12,16.23 U1.30
  Bottom 0.813: I2C.2 191.77,43.18 190.35,41.76 190.35,38.25 SPI.5 | U$1.OUT+ 51.5,23.56 44.45,16.51 40.13,16.51 | 40.13,16.51 J1.2 39.37,16.51 | DZA3.C 86.36,125.09 86.36,123.19 | 86.36,123.19 88.9,120.65 92.08,120.65 DZA1.C | 86.36,123.19 83.82,120.65 77.47,120.65 71.12,127 68.58,127 67.31,125.73 v67.31,99.69 | OLED_LCD.1 v95.25,71.12 95.25,71.28 43.18,71.28 v43.18,71.12 v43.18,33.02 43.18,19.56 40.13,16.51 | U1.30 143.51,16.23 v143.51,16.51 | RL5.2 196.85,19.68 196.85,9.79 189.6,2.54 166.55,2.54 156.21,12.88 U1.30 | U1.30 170.04,16.23 A1.1
12V  (via drill 1 pad 2.03)
  Top 0.813: 144.78,79.38 67.31,79.38 | 67.31,79.38 40.64,79.38 | 40.64,79.38 12.06,79.38 11.43,78.74 v11.43,76.2 | 67.31,79.38 v67.31,76.2 | v11.43,88.9 11.43,99.06 12.7,100.33 OK1.4 | 40.64,79.38 v40.64,71.12 | v151.13,99.69 151.13,80.01 150.5,79.38 144.78,79.38 | 144.78,79.38 v144.78,76.83
  Bottom 0.813: J1.3 10.73,23.43 16.16,23.43 U$1.IN+ 24.83,23.56 27.94,26.67 RL12.1 40.64,29.21 v40.64,33.02 v40.64,71.12 | D2.C 21.59,107.95 21.59,122.02 K1.A1 25.05,125.44 25.4,125.09 R8.1 | D3.C 53.34,107.95 53.34,122.02 K3.A1 57.15,125.83 R7.1 | D2.C 22.86,104.14 19.05,104.14 17.78,102.87 OK1.4 | OK2.4 49.53,102.87 52.07,105.41 D3.C | D4.A 182.88,125.73 179.07,129.54 172.72,129.54 170.18,127 D14.A 173.99,121.92 173.99,115.57 172.72,114.3 156.21,114.3 151.13,109.22 v151.13,99.69 | v11.43,76.2 v11.43,88.9 | D3.C 62.23,111.76 62.23,144.15 58.62,147.75 37.26,147.75 30.48,140.97 30.48,106.68 29.21,105.41 D2.C
A1  (via drill 0.9 pad 2.03, 1 pad 2.03)
  Top 0.813: v139.7,70.74 139.7,73.66 140.34,74.3 153.03,74.3 153.67,74.93 v153.67,86.36
  Bottom 0.406: U1.21 156.21,39.37
  Bottom 0.813: RA11.1 RA12.2 RA13.2 102.87,87.63 104.14,86.36 v153.67,86.36 181.61,86.36 184.15,83.82 v184.15,76.83 | v139.7,70.74 139.7,40.64 141.25,39.09 U1.21
A2  (via drill 1 pad 2.03)
  Top 0.813: v143.51,36.83 143.51,48.1 163.67,68.26 178.59,68.26 181.61,71.28 v181.61,76.83
  Bottom 0.406: U1.22 156.21,36.83
  Bottom 0.813: RA21.1 RA22.2 RA23.2 69.85,85.09 71.12,83.82 179.07,83.82 181.61,81.28 v181.61,76.83 | U1.22 143.78,36.55 v143.51,36.83
AI1
  Bottom 0.813: DZA2.C 88.86,134.66 ANALOG.1 CA1.+ | DZA2.C 93.98,129.54 93.98,127 90.81,123.83 RA11.2 | DZA1.A DZA2.C
AI2
  Bottom 0.813: CA2.+ ANALOG.2 83.86,134.66 DZA4.C | DZA3.A 76.83,133.35 DZA4.C | DZA4.C 77.47,128.27 77.47,125.73 79.38,123.83 RA21.2
COM1
  Bottom 0.813: K1.COM J2.2
COM2
  Bottom 0.813: J3.2 K3.COM
CS
  Bottom 0.406: U1.8 186.97,34.02 SPI.2
D4  (via drill 1 pad 2.03)
  Top 0.813: U1.5 181.61,26.35 174.94,26.35 162.56,13.97 127,13.97 S1.3
  Bottom 0.406: 81.34,13.97 S3.4 | S1.4 113.03,13.93 | 113.03,13.93 S2.3 | S3.3 S2.4 94.04,17.78 88.9,17.78 87.63,19.05 87.63,25.4 86.36,26.67 | S3.4 77.51,13.93 77.47,13.97 77.41,13.97 S4.3 | S4.4 64.83,13.97 62.23,13.97 61.34,14.86 61.34,23.24 64.77,26.67 69.85,26.67 | 69.85,26.67 86.36,26.67 | 86.36,26.67 104.14,26.67 | 104.14,26.67 121.92,26.67 124.46,24.13 124.46,15.24 125.77,13.93 S1.3 130.81,10.02 RA1.2 | S3.4 76.26,19.05 71.12,19.05 71.12,25.4 69.85,26.67 | 113.03,13.93 109.18,17.78 106.68,17.78 105.41,19.05 105.41,25.4 104.14,26.67
  Bottom 0.813: RA1.2 132.49,8.03 132.49,28.35 133.35,29.21 v135.89,29.21 | U1.5 180.87,26.39 172.72,34.54 v172.72,70.48
D12  (via drill 1 pad 2.03)
  Bottom 0.406: U1.27 156.21,24.13
  Bottom 0.813: 156.21,24.13 v143.51,24.13
D13  (via drill 1 pad 2.03)
  Bottom 0.813: U1.28 143.51,21.32 v143.51,21.59
D25  (via drill 1 pad 2.03)  (1 unrouted)
  Bottom 0.406: 155.75,34.02 U1.23
  Bottom 0.813: U1.23 143.51,34.02 v143.51,34.29 | A1.2 172.72,14.61 169.54,11.43 165.1,11.43 RLM35.2
D26  (via drill 1 pad 2.03)
  Bottom 0.813: U1.24 143.51,31.48 v143.51,31.75
GND  (via drill 0.9 pad 2.03, 1 pad 2.03)
  Top 0.813: v82.55,99.69 82.55,82.55 82.87,82.23 | 82.87,82.23 81.92,81.28 9.53,81.28 8.89,80.64 v8.89,76.2 | 82.87,82.23 83.82,81.28 144.78,81.28 146.05,82.55 v146.05,99.69 148.59,102.23 154.94,102.23 v157.48,99.69 | OLED_LCD.2 98.27,63.02 98.27,35.56 102.08,31.75 v135.89,31.75 | R1.2 177.8,84.45 165.1,71.75 v165.1,70.48 | v194.94,38.73 196.85,36.83 v196.85,22.86
  Bottom 0.406: RA2.1 129.54,21.59 130.81,20.32 RA1.1
  Bottom 0.813: U$1.IN- 15.88,6.35 | L5.K 186.69,12.7 186.69,13.97 | 186.69,13.97 186.69,17.78 185.69,18.77 | 185.69,18.77 U1.2 180.16,18.77 165.1,33.84 v165.1,70.48 | 164.1,18.77 CA4.- | U$1.OUT- U$1.IN- | U$1.IN- 13.56,6.76 J1.1 5.08,11.43 2.9,13.61 2.9,25.4 4.17,26.67 L12.K 5.44,26.67 2.9,29.21 2.9,31.75 4.17,33.02 29.21,33.02 30.48,31.75 36.83,31.75 v38.1,33.02 v38.1,71.12 37.97,71.18 13.02,71.18 8.89,75.31 v8.89,76.2 | 72.26,147.32 93.98,147.32 CA1.- | 72.26,147.32 66.04,147.32 66.04,147.19 64.9,146.05 64.9,105.16 R4.2 59.05,100.84 53.47,95.25 43.18,95.25 Q2.E 37.85,97.79 32.77,102.87 | CA1.- DZA2.A 104.14,129.54 104.14,128.13 93.49,117.47 RA12.1 RA13.1 83.19,117.47 RA22.1 RA23.1 v82.55,99.69 | LI2.K CA1.- | LI1.K 134.62,140.97 130.81,144.78 | 130.81,144.78 123.19,144.78 119.38,140.97 LI2.K | RA2.1 128.27,30.48 129.54,31.75 v135.89,31.75 136.21,32.07 139.06,32.07 140.02,31.11 140.02,20.16 141.13,19.05 v143.51,19.05 143.51,18.77 U1.29 163.56,18.77 CA4.- | DZA4.A CA2.- 72.39,147.19 72.26,147.32 | LI2.K 110.9,133.76 110.9,130.81 112.17,129.54 116.84,129.54 120.65,125.73 C4.- 124.46,116.84 R13.2 | C3.- 129.54,118.11 R11.2 | R13.2 124.46,113.03 121.92,110.49 121.92,106.68 120.65,105.41 OK7.2 116.84,103.5 R26.1 | R13.2 R11.2 | R11.2 135.89,107.95 138.43,107.95 | 138.43,107.95 OK6.2 | 138.43,107.95 138.43,107.78 136.61,105.96 136.61,104.86 137.74,103.73 143.92,103.73 146.05,101.6 v146.05,99.69 142.37,99.69 R25.1 | R1.2 177.8,100.33 176.53,99.06 161.29,99.06 R19.2 158.12,101.6 157.48,100.97 v157.48,99.69 | OLED_LCD.2 v97.79,71.12 | R5.1 36.73,130.22 32.77,126.25 32.77,102.87
  Bottom 0.813: R3.2 4.83,128.27 4.83,98.55 5.59,97.79 Q1.E 11.43,95.25 22.86,95.25 26.67,99.06 26.67,101.6 R2.2 32.77,102.87 | 130.81,144.78 132.08,146.05 155.19,146.05 157.48,143.76 R22.2 160.02,146.05 185.67,146.05 187.96,143.76 R21.2 | SPI.1 193.04,26.67 | 193.04,26.67 193.04,26.04 185.78,18.77 185.69,18.77 | I2C.1 v194.94,38.73 | 193.04,26.67 v196.85,22.86 | 186.69,13.97 179.07,13.97 175.9,10.79 RLM35.1 175.9,15.73 A1.3 175.26,17.78 172.72,20.32 165.1,20.32 CA4.- | 164.47,19.68 CA4.-
  pour Bottom: 2.03,148.59 197.23,148.59 197.23,1.78 2.03,1.78
IN1
  Bottom 0.813: D7.A 135.89,137.16 130.81,137.16 129.5,138.47 DIGITAL-IN.1
IN2
  Bottom 0.813: DIGITAL-IN.2 119.38,135.85 119.38,133.35 118.11,132.08 D8.A
MISO
  Bottom 0.406: U1.10 186.97,39.09 SPI.6
MOSI
  Bottom 0.406: U1.15 194.59,51.8 196.85,49.53 196.85,34.29 195.58,33.02 SPI.3
N$1
  Bottom 0.813: R4.1 55.37,88.14 52.07,91.44 OK2.2
N$2
  Bottom 0.406: OK1.2 20.32,91.44
  Bottom 0.813: OK1.2 20.32,90.17 21.59,88.9 26.67,88.9 R2.1
N$3
  Bottom 0.813: R3.1 8,107.06 6.35,105.41 6.35,101.6 7.62,100.33 Q1.B 12.06,100.33 14.61,97.79 19.05,97.79 20.32,99.06 OK1.3
N$4  (1 unrouted)
  Bottom 0.813: 44.8,125.38 48.26,121.92 48.26,107.95 D3.A 41.91,105.41 40.64,104.14 Q2.C | K3.A2 48.51,125.48 50.16,123.83 52.07,123.83 53.34,125.09 53.34,144.78 51.79,146.33 41.19,146.33 39.6,144.74 39.6,144.25 LNO2.K
N$5
  Bottom 0.406: RA5.1 RA4.2 85.09,17.78 85.09,10.16 83.86,8.93 S3.2
  Bottom 0.813: S3.2 S3.1
N$6
  Bottom 0.813: R5.2 36.83,102.87 39.37,100.33 Q2.B 45.72,100.33 48.9,97.16 OK2.3
N$7
  Bottom 0.813: R7.2 46.99,132.08 48.26,133.35 48.26,142.88 46.99,144.15 42.04,144.15 LNO2.A
N$8
  Bottom 0.406: RA4.1 RA3.2 101.6,19.05 101.6,11.43 99.1,8.93 S2.2
  Bottom 0.813: S2.2 S2.1
N$9
  Bottom 0.406: RA3.1 RA2.2 118.11,19.05 118.11,11.43 115.61,8.93 S1.2
  Bottom 0.813: S1.2 S1.1 | S1.1 126.96,8.93 127,8.89 126.94,8.89 S1.1
N$10
  Bottom 0.813: LNO1.A 10.79,144.65 10.79,144.78 15.88,144.78 16.51,144.15 16.51,133.35 15.24,132.08 R8.2
N$11
  Bottom 0.813: Q1.C 11.43,105.41 D2.A 13.97,107.31 17.14,110.49 17.14,121.39 K1.A2 16.12,125.48 18.41,123.19 20.32,123.19 21.59,124.46 21.59,146.05 20.32,147.32 7.62,147.32 7.14,146.84 7.14,144.67 6.99,144.52 LNO1.K
N$14
  Bottom 0.813: L12.A RL12.2
N$15
  Bottom 0.813: OK3.1 180.34,109.22 D1.C
N$16
  Bottom 0.813: OK3.2 182.88,104.14 185.42,101.6 R1.1
N$17  (via drill 1 pad 2.03)
  other vias: 64.77,76.2
N$18
  Bottom 0.813: D4.C 180.34,123.19 OK3.4
N$19
  Bottom 0.813: RLI1.1 144.78,128.27 R12.2 143.51,124.46 139.7,120.65 C3.+ 142.24,115.57 R11.1 143.51,113.03 143.51,106.68 142.24,105.41 OK6.1
N$20
  Bottom 0.813: D7.C R12.1
N$21
  Bottom 0.813: RLI2.1 109.22,128.27 110.49,127 R14.2 111.76,123.19 114.3,120.65 C4.+ 111.76,116.84 R13.1 111.76,109.22 113.03,107.95 OK7.1
N$22
  Bottom 0.813: D8.C R14.1
N$23
  Bottom 0.813: L5.A RL5.1
N$24
  Bottom 0.813: LI2.A RLI2.2
N$25  (via drill 1 pad 2.03)
  Bottom 0.406: U1.16 157.75,51.8 158.75,50.8 158.75,29.21 CA4.+
  Bottom 0.813: U1.16 153.67,51.8 152.4,53.06 v152.4,70.48
N$26
  Bottom 0.813: D13.C 167.64,106.68 166.37,107.95 OK10.1
N$27
  Bottom 0.813: OK10.2 172.37,111.76 174.14,109.99 174.14,103.02 172.72,101.6 R19.1
N$28  (via drill 1 pad 2.03)
  other vias: 62.23,76.2
N$29
  Bottom 0.813: LI1.A RLI1.2
N$30
  Bottom 0.813: LO1.K 187.96,135.89 R21.1
N$31
  Bottom 0.813: R22.1 157.48,135.89 LO2.K
N$32
  Bottom 0.406: RA5.2 67.35,17.74 67.35,13.88 67.31,13.84 67.31,11.37 S4.2
  Bottom 0.813: RA6.1 131.17,2.9 78.38,2.9 72.35,8.93 | S4.2 72.35,8.93 | 72.35,8.93 S4.1
N$33  (via drill 1 pad 2.03)
  other vias: 139.7,76.83
N$34  (via drill 1 pad 2.03)
  other vias: 142.24,76.83
N$52
  Bottom 0.813: D14.C 160.02,121.92 162.56,119.38 OK10.4
NC1
  Bottom 0.813: J2.3 27.94,137.16 27.94,116.17 K1.NC
NC2
  Bottom 0.813: J3.3 59.69,137.16 59.69,116.17 K3.NC
NO1
  Bottom 0.813: J2.1 9.78,136.78 9.78,115.95 12.45,113.28 K1.NO
NO2
  Bottom 0.813: J3.1 40.64,135.89 40.64,116.84 44.2,113.28 K3.NO
OUT1
  Bottom 0.813: OK3.3 190.63,119.38 193.04,121.79 193.04,125.73 190.63,128.14 184.28,128.14 175.26,137.16 175.26,140.93 DIGITAL-OUT.1 177.76,143.51 LO1.A
OUT2
  Bottom 0.813: OK10.3 170.18,119.38 170.59,119.79 170.59,121.51 166.12,125.98 166.12,131.83 170.22,135.93 DIGITAL-OUT.2 170.22,141.95 168.66,143.51 LO2.A
R1  (via drill 1 pad 2.03)
  Top 0.813: v194.31,76.83 194.31,73.03 177.48,56.2 177.48,49.37 157.16,29.05 156.21,29.05 U1.25
  Bottom 0.406: U1.25 156.49,29.21
  Bottom 0.813: D1.A 193.04,106.68 194.31,105.41 v194.31,76.83 | U1.25 143.51,28.93 v143.51,29.21
R2  (via drill 0.9 pad 2.03, 1 pad 2.03)
  Top 0.813: v191.77,76.83 191.77,73.66 162.56,44.45 162.56,40.64 v160.66,38.73
  Bottom 0.406: U1.26 156.49,26.67
  Bottom 0.813: D13.A 156.21,106.68 154.31,104.78 154.31,95.89 156.21,93.98 186.69,93.98 191.77,88.9 v191.77,76.83 | v143.51,26.67 156.21,26.67 U1.26 156.53,26.19 157,25.72 158.43,25.72 162.08,22.07 165.58,22.07 166.85,23.34 166.85,26.67 160.66,32.86 v160.66,38.73
RR1  (via drill 1 pad 2.03)
  Top 0.813: v167.64,70.48 167.64,71.75 172.72,76.83 v176.53,76.83
  Bottom 0.406: U1.3 181.34,21.59
  Bottom 0.813: OK1.1 17.78,83.82 22.23,79.38 174.62,79.38 176.53,77.47 v176.53,76.83 | U1.3 180.16,21.32 167.64,33.84 v167.64,70.48
RR2  (via drill 1 pad 2.03)
  Top 0.813: v170.18,70.48 170.18,71.75 172.28,73.85 177.86,73.85 179.07,75.06 v179.07,76.83
  Bottom 0.406: U1.4 181.34,24.13
  Bottom 0.813: v179.07,76.83 179.07,80.01 177.8,81.28 52.07,81.28 49.53,83.82 OK2.1 | U1.4 180.87,23.86 170.18,34.54 v170.18,70.48
RX0
  Bottom 0.406: UART.2 181.88,44.72 181.61,44.45 U1.12
RX2
  Bottom 0.406: U1.6 182.16,29.48 UART2.2
S1  (via drill 0.9 pad 2.03, 1 pad 2.03)
  Top 0.813: v144.78,70.48 144.78,72.09 145.56,72.87 157.43,72.87 158.12,73.55 v158.12,91.44
  Bottom 0.406: U1.19 156.21,44.45
  Bottom 0.813: v189.23,76.83 189.23,87.63 185.42,91.44 v158.12,91.44 131.06,91.44 129.54,92.96 R25.2 | 156.21,44.45 146.05,44.45 144.78,45.72 v144.78,70.48 | R25.2 130.68,99.82 | OK6.3 132.33,107.95 134.87,105.41 134.87,101.22 133.48,99.82 R25.2
S2  (via drill 1 pad 2.03)
  Top 0.813: v186.69,76.83 186.69,73.66 160.66,47.62 160.66,43.97 158.43,41.75 156.21,41.75 U1.20
  Bottom 0.406: U1.20 156.21,41.91
  Bottom 0.813: v186.69,76.83 186.69,86.36 184.15,88.9 126.36,88.9 125.73,89.53 R26.2 125.73,104.14 OK7.3 | v142.24,70.61 142.24,43.18 143.78,41.63 U1.20
SCK
  Bottom 0.406: U1.9 186.97,36.55 SPI.4
SCL  (via drill 1 pad 2.03)
  Bottom 0.406: I2C.4 183.06,48.26 183.03,48.29 182.57,48.29 U1.14
  Bottom 0.813: OLED_LCD.3 v100.33,71.12 100.33,72.87 102.23,74.77 175.26,74.77 177.8,72.23 v177.8,70.48 177.8,50.8 179.07,49.53 181.34,49.53 U1.14
SDA  (via drill 1 pad 2.03)
  Bottom 0.406: I2C.3 190.5,45.72 189.23,44.45 189.23,43.18 187.69,41.63 U1.11 | U1.11 181.34,41.91 | U1.11 179.34,41.63
  Bottom 0.813: OLED_LCD.4 v102.87,71.12 103.19,71.28 104.74,72.83 174.09,72.83 v175.26,70.48 175.26,44.45 178.07,41.63 U1.11
TX0
  Bottom 0.406: UART.1 U1.13
TX2
  Bottom 0.406: UART2.1 U1.7
VN  (via drill 1 pad 2.03)
  Bottom 0.406: 156.49,46.99 U1.18
  Bottom 0.813: v147.32,70.48 147.32,48.26 148.87,46.72 U1.18
VP  (via drill 1 pad 2.03)
  Bottom 0.813: v149.86,70.48 149.86,50.52 151.13,49.26 U1.17
(copper drawn outside any net)
  shapes: Bottom area x112

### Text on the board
Bottom: ISOESP32 VER 0.1 / AGROVOLTAIC / BY ALMUZKY & SALMAN
tPlace: ISOLATION SPACE | CUSTOM SPACE | MICROCONTROLLER | DISPLAY SPACE | POWER DISTRIBUTION | BUTTON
